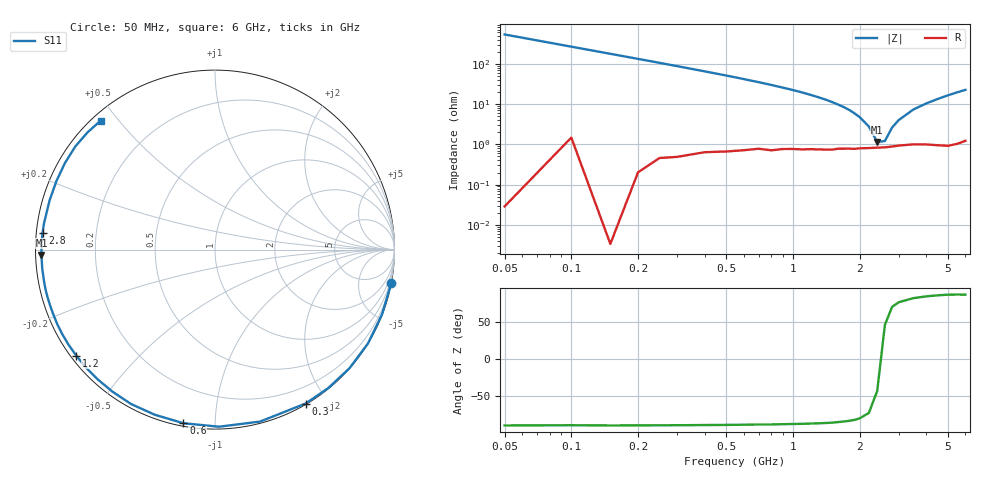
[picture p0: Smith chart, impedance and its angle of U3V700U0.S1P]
! SIEMENS Discrete & RF Semiconductors
! BBY53-02W
! Si Tuning Diode in SCD-80
! VR = 0.7 V
! S-Parameters:  September  1997
# GHz  S  MA  R  50
!  f  S11
! GHz  MAG  ANG
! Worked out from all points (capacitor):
!   34 points, 50 MHz to 6 GHz, reference 50 ohm
!   read as one part to ground: C = 5.98 pF near 50 MHz
!   lowest |Z| = 1.14 ohm at 2.4 GHz (marker M1)
!   series resonance near 2.495 GHz, so ESL is about 680 pH
!   S11 on the Smith chart (normalised r, x): 50 MHz: 0, -11; 300 MHz: 0.01, -1.75; 600 MHz: 0.01, -0.83; 1.2 GHz: 0.02, -0.34; 2.8 GHz: 0.02, +0.05; 6 GHz: 0.02, +0.45
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0.05  1 -10.7
0.1  0.998 -21.3
0.15  1 -31.6
0.2  0.999 -41.4
0.25  0.9967 -50.7
0.3  0.9952 -59.5
0.4  0.9905 -75.3
0.5  0.9871 -88.7
0.6  0.9833 -100.3
0.7  0.9793 -110.1
0.8  0.9792 -118.5
0.9  0.976 -125.8
1  0.9747 -132.0
1.1  0.9743 -137.5
1.2  0.9731 -142.6
1.3  0.9729 -147.0
1.4  0.9725 -151.0
1.6  0.9704 -158.1
1.9  0.9699 -166.8
2.2  0.9683 -173.9
2.4  0.9675 -178.2
2.8  0.9654 174.4
3.5  0.9615 163.4
4  0.9626 156.6
4.5  0.9651 150.1
5  0.9674 143.6
5.5  0.965 137.4
6  0.9601 131.6
